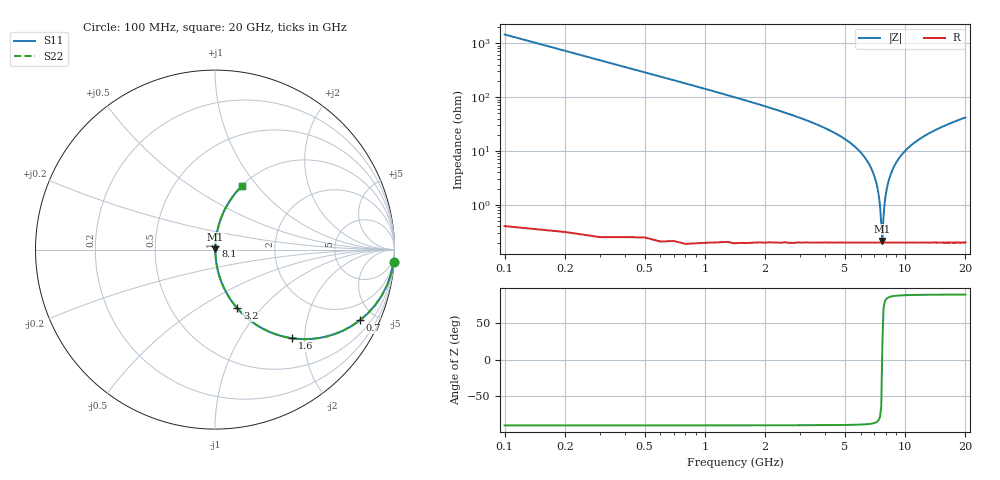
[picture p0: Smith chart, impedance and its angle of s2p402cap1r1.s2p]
! AVX Thin Film Operation		Date: April 2003
! Description: Accu-P® Series, Thin Film, SMD, RF Capacitor
! Part Number: 04021J1R1ABS
! 50 MHz  -  20 GHz
! Serial Measurements
# hz S db R 50
!	S11		S21		S12		S22
!	dB	Phase	dB	Phase	dB	Phase	dB	Phase
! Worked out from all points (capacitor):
!   200 points, 100 MHz to 20 GHz, reference 50 ohm
!   read as one part in series: C = 1.1 pF near 200 MHz
!   lowest |Z| = 215 mohm at 7.7 GHz (marker M1)
!   series resonance near 7.684 GHz, so ESL is about 390 pH
!   S11 on the Smith chart (normalised r, x): 100 MHz: 1, -29; 700 MHz: 1.00, -4.10; 1.6 GHz: 1.00, -1.73; 3.2 GHz: 1.00, -0.75; 8.1 GHz: 1.00, +0.04; 20 GHz: 1.00, +0.84
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1e8  -0.02 -4.0  -23.23 86.0  -23.23 86.0  -0.02 -4.0
2e8  -0.08 -7.9  -17.26 82.1  -17.26 82.1  -0.08 -7.9
3e8  -0.18 -11.7  -13.84 78.2  -13.84 78.2  -0.18 -11.7
7e8  -0.93 -26.0  -7.17 64.0  -7.17 64.0  -0.93 -26.0
1.6e9  -3.69 -49.1  -2.44 40.8  -2.44 40.8  -3.69 -49.1
3.2e9  -9.13 -69.2  -0.58 20.4  -0.58 20.4  -9.13 -69.2
3.5e9  -10.15 -71.5  -0.46 18.1  -0.46 18.1  -10.15 -71.5
5.6e9  -18.41 -82.2  -0.08 6.9  -0.08 6.9  -18.41 -82.2
6.8e9  -26.74 -84.9  -0.03 2.6  -0.03 2.6  -26.74 -84.9
7.2e9  -32.20 -83.9  -0.02 1.4  -0.02 1.4  -32.20 -83.9
7.4e9  -36.89 -81.2  -0.02 0.8  -0.02 0.8  -36.89 -81.2
7.5e9  -40.60 -77.1  -0.02 0.5  -0.02 0.5  -40.60 -77.1
7.7e9  -53.38 21.2  -0.02 -0.0  -0.02 -0.0  -53.38 21.2
7.8e9  -44.48 70.2  -0.02 -0.3  -0.02 -0.3  -44.48 70.2
7.9e9  -39.49 78.5  -0.02 -0.6  -0.02 -0.6  -39.49 78.5
8.1e9  -34.02 83.1  -0.02 -1.1  -0.02 -1.1  -34.02 83.1
8.4e9  -29.48 84.7  -0.02 -1.9  -0.02 -1.9  -29.48 84.7
8.8e9  -25.83 84.8  -0.03 -2.9  -0.03 -2.9  -25.83 84.8
1.01e10  -19.70 83.0  -0.06 -5.9  -0.06 -5.9  -19.70 83.0
1.34e10  -13.36 77.1  -0.22 -12.4  -0.22 -12.4  -13.36 77.1
1.67e10  -10.27 71.8  -0.45 -17.9  -0.45 -17.9  -10.27 71.8
2e10  -8.29 67.1  -0.71 -22.6  -0.71 -22.6  -8.29 67.1
